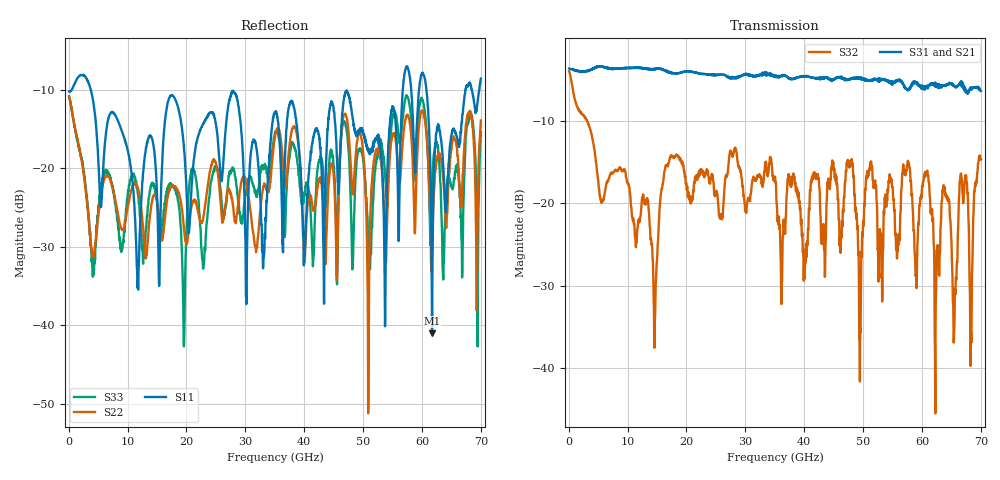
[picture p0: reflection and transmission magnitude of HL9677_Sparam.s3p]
! 5/24/2024 9:44:19 AM
! H:\PROTOTYPE_DATA\WILKINSON\PROTO1-LID.S3P
! CHANNEL.1
! TR.MEASUREMENT
! CORRECTED.DATA
# GHZ S RI R 50.0
! FREQ.GHZ  S11RE  S11IM  S12RE  S12IM  S13RE  S13IM
!  S21RE  S21IM  S22RE  S22IM  S23RE  S23IM
!  S31RE  S31IM  S32RE  S32IM  S33RE  S33IM
!; PortSelection: Port_123
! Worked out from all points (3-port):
!   1999 points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, 70 MHz to 70 GHz, reference 50 ohm
!   strongest paths, dB at 70 MHz, 17.54 GHz, 35.03 GHz, 52.53 GHz, 70 GHz:
!     S31: -3.7, -4.3, -4.6, -5.0, -6.4
!     S21: -3.7, -4.3, -4.8, -5.1, -6.7
!     S32: -4.0, -14.4, -16.8, -25.5, -14.7
!   lowest |S11| = -41.0 dB at 61.7 GHz (marker M1), VSWR 1.02, Z = 50.8 + j0.395 ohm
!   |S11| at or under -10 dB: 3.756 GHz to 56.74 GHz (52.98 GHz wide, 175 % of centre); 58.16 GHz to 59.5 GHz (1.341 GHz wide, 2.28 % of centre); 60.75 GHz to 67.37 GHz (6.62 GHz wide, 10.3 % of centre)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
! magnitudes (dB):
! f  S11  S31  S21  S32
! 70 MHz  -10.2  -3.7  -3.7  -4.0
! 4.165 GHz  -11.5  -3.7  -3.8  -12.7
! 14.6 GHz  -18.3  -3.8  -3.8  -35.5
! 19.57 GHz  -17.4  -4.1  -4.1  -16.1
! 35.03 GHz  -12.9  -4.6  -4.8  -16.8
! 49.49 GHz  -15.2  -4.8  -5.0  -36.6
! 50.89 GHz  -17.9  -5.1  -5.2  -16.5
! 60.16 GHz  -7.9  -5.9  -6.1  -17.4
! 61.7 GHz  -41.0  -5.5  -5.8  -20.7
! 70 GHz  -8.6  -6.4  -6.7  -14.7
